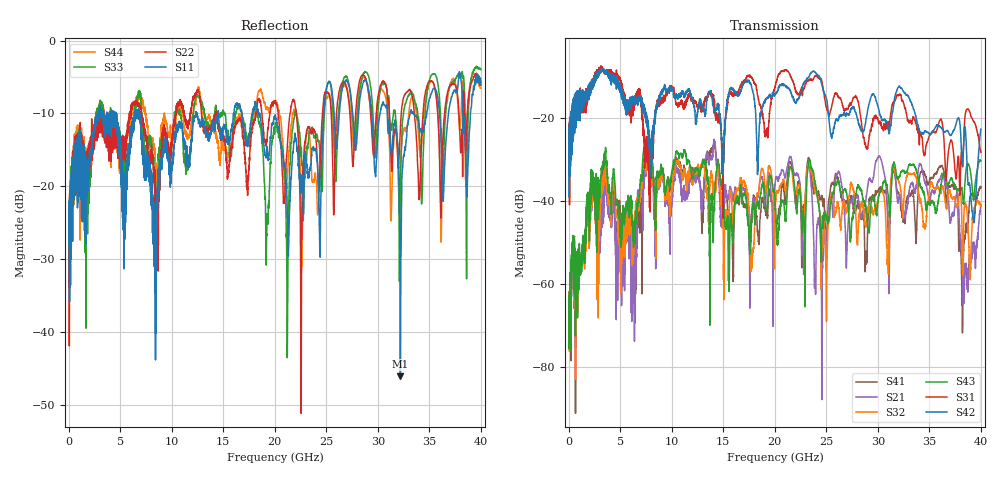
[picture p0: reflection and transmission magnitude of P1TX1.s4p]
!Agilent Technologies,N5245A,MY49151084,A.09.20.08
!Agilent N5245A: A.09.20.08
!Date: Thursday, March 01, 2012 14:01:14
!Correction: S11(Full 4 Port(1,2,3,4))
!S12(Full 4 Port(1,2,3,4))
!S13(Full 4 Port(1,2,3,4))
!S14(Full 4 Port(1,2,3,4))
!S21(Full 4 Port(1,2,3,4))
!S22(Full 4 Port(1,2,3,4))
!S23(Full 4 Port(1,2,3,4))
!S24(Full 4 Port(1,2,3,4))
!S31(Full 4 Port(1,2,3,4))
!S32(Full 4 Port(1,2,3,4))
!S33(Full 4 Port(1,2,3,4))
!S34(Full 4 Port(1,2,3,4))
!S41(Full 4 Port(1,2,3,4))
!S42(Full 4 Port(1,2,3,4))
!S43(Full 4 Port(1,2,3,4))
!S44(Full 4 Port(1,2,3,4))
!S4P File: Measurements: <S11,S12,S13,S14>,
!<S21,S22,S23,S24>,
!<S31,S32,S33,S34>,
!<S41,S42,S43,S44>:
# Hz S  dB  R 50
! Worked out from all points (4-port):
!   3996 points, 50 MHz to 40 GHz, reference 50 ohm
!   strongest paths, dB at 50 MHz, 10.04 GHz, 20.03 GHz, 30.02 GHz, 40 GHz:
!     S42: -24.9, -12.9, -14.3, -17.1, -22.6
!     S31: -23.7, -12.9, -12.5, -20.4, -28.2
!     S43: -61.7, -32.5, -39.8, -40.1, -30.2
!     S32: -61.8, -36.5, -44.7, -39.6, -41.2
!     S21: -71.6, -39.9, -36.0, -29.4, -40.9
!     S41: -63.7, -33.9, -44.1, -37.6, -36.7
!   lowest |S11| = -46.0 dB at 32.19 GHz (marker M1), VSWR 1.01, Z = 50.5 - j0.0458 ohm
!   |S11| at or under -10 dB: start of sweep to 2.8 GHz; 6.871 GHz to 12.34 GHz (5.47 GHz wide, 56.9 % of centre); 18.55 GHz to 24.76 GHz (6.209 GHz wide, 28.7 % of centre)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
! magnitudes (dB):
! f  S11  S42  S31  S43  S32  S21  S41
! 50 MHz  -23.6  -24.9  -23.7  -61.7  -61.8  -71.6  -63.7
! 3.52 GHz  -12.5  -8.7  -9.1  -28.1  -32.6  -36.1  -31.9
! 6.35 GHz  -10.6  -16.5  -16.7  -46.5  -47.3  -48.9  -53.0
! 7.82 GHz  -16.8  -23.0  -38.4  -26.9  -28.0  -26.0  -25.0
! 32.19 GHz  -46.0  -12.6  -14.2  -33.3  -36.9  -38.6  -40.4
! 39.27 GHz  -6.4  -44.1  -20.7  -39.6  -42.4  -50.6  -38.8
! 40 GHz  -6.1  -22.6  -28.2  -30.2  -41.2  -40.9  -36.7
